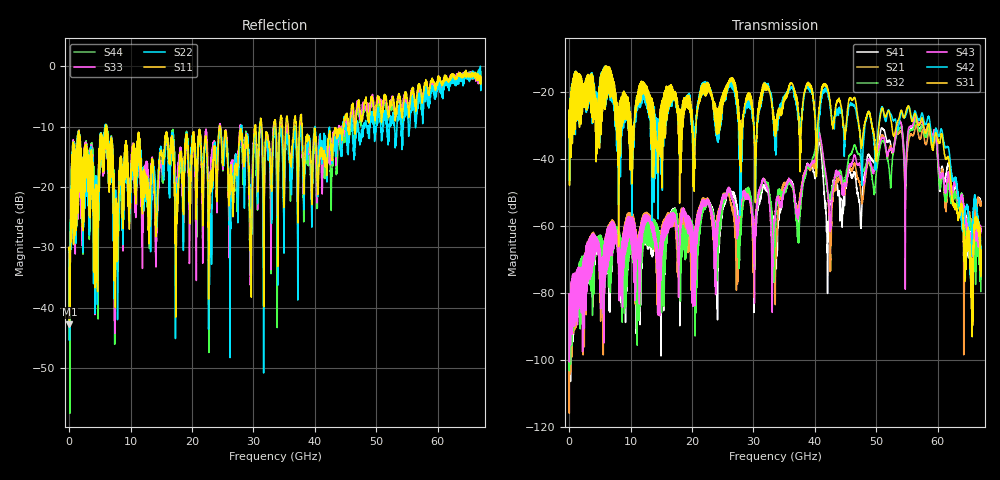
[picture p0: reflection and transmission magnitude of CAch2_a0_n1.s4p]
!Agilent Technologies,N5247A,US51170199,A.09.90.13
!Agilent N5247A: A.09.90.13
!Date: Wednesday, October 17, 2018 17:07:10
!Correction: S11(Full 4 Port(1,2,3,4))
!S12(Full 4 Port(1,2,3,4))
!S13(Full 4 Port(1,2,3,4))
!S14(Full 4 Port(1,2,3,4))
!S21(Full 4 Port(1,2,3,4))
!S22(Full 4 Port(1,2,3,4))
!S23(Full 4 Port(1,2,3,4))
!S24(Full 4 Port(1,2,3,4))
!S31(Full 4 Port(1,2,3,4))
!S32(Full 4 Port(1,2,3,4))
!S33(Full 4 Port(1,2,3,4))
!S34(Full 4 Port(1,2,3,4))
!S41(Full 4 Port(1,2,3,4))
!S42(Full 4 Port(1,2,3,4))
!S43(Full 4 Port(1,2,3,4))
!S44(Full 4 Port(1,2,3,4))
!S4P File: Measurements: <S11,S12,S13,S14>,
!<S21,S22,S23,S24>,
!<S31,S32,S33,S34>,
!<S41,S42,S43,S44>:
# Hz S  dB  R 50
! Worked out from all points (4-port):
!   6701 points, 10 MHz to 67 GHz, reference 50 ohm
!   strongest paths, dB at 10 MHz, 16.76 GHz, 33.51 GHz, 50.25 GHz, 67 GHz:
!     S31: -33.4, -22.4, -29.8, -33.2, -70.3
!     S42: -33.5, -22.9, -28.9, -31.7, -68.5
!     S43: -80.2, -60.0, -57.7, -37.2, -60.1
!     S32: -90.8, -56.5, -63.8, -40.6, -79.5
!     S21: -84.1, -59.8, -68.8, -39.9, -54.0
!     S41: -80.2, -56.4, -60.0, -37.6, -52.8
!   lowest |S11| = -42.7 dB at 69.99 MHz (marker M1), VSWR 1.01, Z = 50.2 + j0.712 ohm
!   |S11| at or under -10 dB: start of sweep to 5.98 GHz; 6.102 GHz to 24.48 GHz (18.37 GHz wide, 120 % of centre); 37.92 GHz to 44.61 GHz (6.695 GHz wide, 16.2 % of centre)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
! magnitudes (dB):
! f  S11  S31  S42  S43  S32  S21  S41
! 10 MHz  -30.4  -33.4  -33.5  -80.2  -90.8  -84.1  -80.2
! 69.99 MHz  -42.7  -32.7  -32.6  -93.3  -92.7  -91.4  -94.5
! 33.47 GHz  -8.9  -30.7  -32.1  -57.4  -61.7  -69.7  -59.9
! 40.69 GHz  -16.5  -24.5  -27.9  -32.1  -31.4  -33.7  -34.8
! 42.09 GHz  -13.5  -19.3  -20.0  -49.5  -50.5  -51.4  -62.8
! 56.44 GHz  -7.0  -27.1  -26.2  -27.3  -28.0  -29.8  -28.1
! 67 GHz  -2.9  -70.3  -68.5  -60.1  -79.5  -54.0  -52.8
